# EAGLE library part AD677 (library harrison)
Analog Devices AD677 16-bit +/-10V ADC
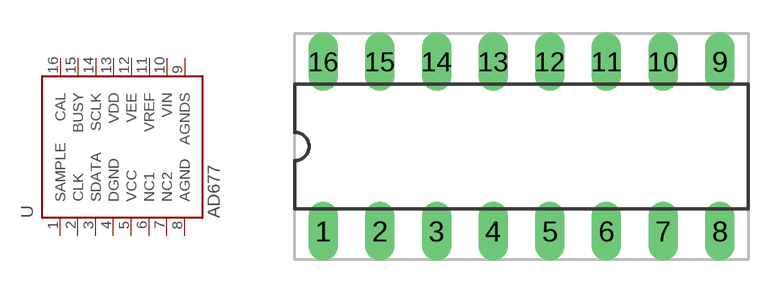
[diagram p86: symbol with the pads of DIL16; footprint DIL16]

Designator prefix U

## AD677-DIP  [DIL16]
1  SAMPLE  in
2  CLK  in
3  SDATA  out
4  DGND  pwr
5  VCC  pwr
6  NC1  nc
7  NC2  nc
8  AGND  pwr
9  AGNDS  in
10  VIN  in
11  VREF  in
12  VEE  pwr
13  VDD  pwr
14  SCLK  out
15  BUSY  out
16  CAL  in

## Footprint DIL16 (pad centres in mm)
drill 0.813 long: 1 -8.89,-3.81; 2 -6.35,-3.81; 3 -3.81,-3.81; 4 -1.27,-3.81; 5 1.27,-3.81; 6 3.81,-3.81; 7 6.35,-3.81; 8 8.89,-3.81; 9 8.89,3.81; 10 6.35,3.81; 11 3.81,3.81; 12 1.27,3.81; 13 -1.27,3.81; 14 -3.81,3.81; 15 -6.35,3.81; 16 -8.89,3.81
